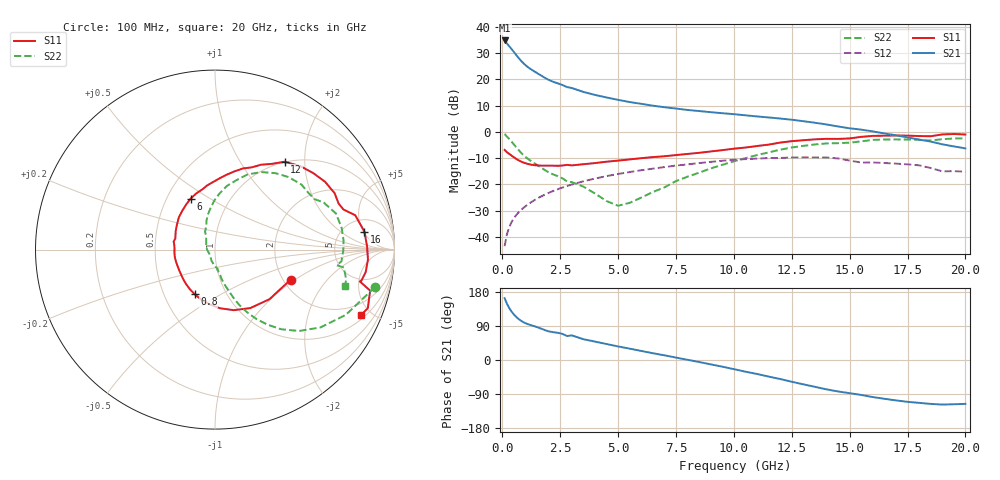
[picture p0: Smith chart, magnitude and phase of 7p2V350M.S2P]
! Infineon Technologies  Discrete & RF Semiconductors
! bfp620
! VCE =  2.3 V,  IC =  50 mA
! Common Emitter S-Parameters:  Sep 2002
# GHz  S  MA  R  50
!  f  S11  S21  S12  S22
! GHz  MAG  ANG  MAG  ANG  MAG  ANG  MAG  ANG
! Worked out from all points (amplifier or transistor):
!   59 points, 100 MHz to 20 GHz, reference 50 ohm
!   highest |S21| = 34.9 dB at 100 MHz (marker M1)
!   |S21| within 3 dB of that: start of sweep to 374.4 MHz
!   unconditionally stable (mu >= 1): 2.603 GHz to 9.826 GHz; 17.2 GHz to end of sweep
!   at 1 GHz: K = 0.86, MSG = 26.9 dB, |S12| = -28.4 dB
!   at 5.5 GHz: K = 1.04, MAG = 12.2 dB, |S12| = -15.3 dB
!   at 20 GHz: K = 1.24, MAG = 1.5 dB, |S12| = -15.2 dB
!   S11 on the Smith chart (normalised r, x): 100 MHz: 2.19, -0.92; 800 MHz: 0.71, -0.38; 6 GHz: 0.66, +0.42; 12 GHz: 0.99, +1.59; 16 GHz: 7.77, +5.28; 20 GHz: 1.22, -4.34
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0.1  0.4533 -21.7  55.54 163.3  0.0066 68.4  0.9144 -13.3
0.2  0.4105 -42.3  48.6 148.5  0.0111 68.6  0.8146 -26.5
0.3  0.3806 -58.9  43.09 136.9  0.0152 67.7  0.7304 -36.4
0.4  0.3533 -72.8  38.1 127.7  0.019 66.8  0.6516 -44.1
0.5  0.3279 -85.1  33.51 120.1  0.0225 66.0  0.5777 -50.2
0.6  0.3056 -96.1  29.41 113.8  0.0258 65.4  0.5109 -55.0
0.7  0.2874 -106.0  25.9 108.4  0.029 64.9  0.453 -59.0
0.8  0.2729 -114.7  22.99 103.9  0.0321 64.6  0.4045 -62.1
0.9  0.2615 -122.3  20.65 100.2  0.0351 64.3  0.365 -64.6
1.1  0.245 -134.4  17.3 94.8  0.0411 63.6  0.3073 -67.9
1.4  0.2312 -148.3  14.13 88.9  0.0502 62.5  0.2504 -71.1
1.9  0.2275 -167.8  10.4 77.6  0.0655 59.6  0.18 -76.4
2.8  0.2349 168.8  7.15 63.1  0.0929 52.7  0.1133 -83.3
3.5  0.2417 155.0  5.801 54.9  0.1141 46.6  0.0905 -90.9
6  0.3149 115.4  3.43 23.9  0.1854 23.2  0.0557 151.4
7  0.3428 101.9  2.956 12.4  0.213 13.7  0.0872 124.7
10.5  0.5026 65.8  2.071 -30.8  0.3025 -25.5  0.315 85.2
12  0.6249 51.6  1.799 -50.2  0.3179 -43.1  0.4571 66.5
13.5  0.7205 31.6  1.495 -70.8  0.3255 -62.0  0.5756 44.6
16  0.8386 6.9  1.022 -97.8  0.2607 -86.1  0.7037 16.6
17  0.8541 -3.7  0.861 -106.6  0.2481 -94.1  0.7181 4.1
20  0.8917 -24.2  0.484 -115.8  0.1743 -103.4  0.7534 -15.8
